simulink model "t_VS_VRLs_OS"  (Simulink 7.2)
settings: Solver=ode3  StartTime=0.0  StopTime=0.02  FixedStep=1e-5  RelTol=1e-3

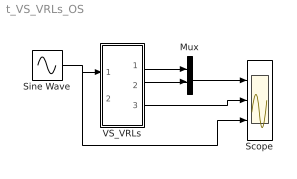
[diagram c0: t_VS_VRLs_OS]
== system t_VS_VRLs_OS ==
  Mux : Mux  Inputs=2
  Scope : Scope  NumInputPorts=3
  Sine Wave : Sin  Amplitude=230*sqrt(2)  Frequency=1000*pi  SampleTime=0
  VS_VRLs : Subsystem  mask(VS_VRLs_OS){R=1, L=1e-3, IL0=0, RLp=1e6}
      mask prompts: R "Output Resistance"; L "Output Inductance"; IL0 "Initial Inductor Current"; RLp "Ind. Parallel Res"
      mask help: Open source VS_VRL_Series Input Vector: u[0]= Vs, Source Voltage u[1]= E, Load Voltage Output Vector: y[0]=IL, Load current y[1]=VL, Inductance Voltage y[2]=VR, Resistance Voltage Parameter Vector: p[0]=R p[1]=L p[2]=IL0
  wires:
  Sine Wave/1 -> VS_VRLs/1(v), Scope/3
  VS_VRLs/1(iL) -> Mux/1
  VS_VRLs/2(vL) -> Mux/2
  Mux/1 -> Scope/1
  VS_VRLs/3(vR) -> Scope/2

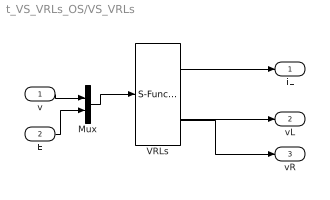
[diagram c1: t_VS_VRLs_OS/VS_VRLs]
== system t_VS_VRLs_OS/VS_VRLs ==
  v : Inport
  E : Inport  Port=2
  Mux : Mux  Inputs=2
  VRLs : S-Function  FunctionName=s_VS_VRLs_OS  Parameters=[R, L, IL0, RLp]  EnableBusSupport=off
  iL : Outport
  vL : Outport  Port=2
  vR : Outport  Port=3
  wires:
  Mux/1 -> VRLs/1
  E/1 -> Mux/2
  v/1 -> Mux/1
  VRLs/1 -> iL/1
  VRLs/2 -> vL/1
  VRLs/3 -> vR/1
